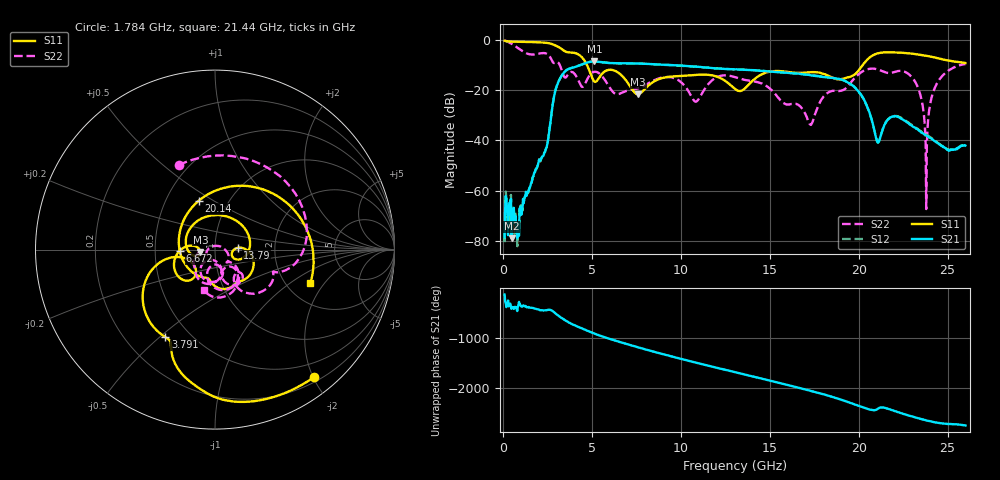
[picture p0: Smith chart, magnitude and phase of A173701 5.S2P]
!  2-Port S-parameters saved by WinCal
! VAR MeasName=S-Parameters (CALIBRATED_DATA) read from VNA (N5245A)
! VAR MeasDate=2017-6-7 10:28:45
! VAR NAME=A173701 5
! VAR FILENAME=A173701 5.S2P
! VAR DATE=2017-6-7 10:28:45
! VAR PHYS_PORTS=1,2
# Hz S DB R 50
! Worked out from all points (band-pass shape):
!   801 points, 100 MHz to 26 GHz, reference 50 ohm
!   highest |S21| = -8.61 dB at 5.151 GHz (marker M1); lowest = -79.0 dB at 488.5 MHz (marker M2)
!   |S21| within 3 dB of the highest: 3.696 GHz to 12.6 GHz (8.906 GHz wide, 109 % of centre)
!   lowest |S11| = -21.6 dB at 7.611 GHz (marker M3), VSWR 1.18, Z = 42.4 - j1.08 ohm
!   |S11| at or under -10 dB: 4.729 GHz to 20.23 GHz (15.5 GHz wide, 124 % of centre)
!   |S22| runs from -67.3 to -0.2 dB; largest |S21 - S12| = 0.0043
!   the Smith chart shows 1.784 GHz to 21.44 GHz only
!   S11 on the Smith chart (normalised r, x): 1.784 GHz: 0.27, -2.01; 3.791 GHz: 0.37, -0.52; 6.672 GHz: 0.67, -0.01; 13.79 GHz: 1.29, +0.03; 20.14 GHz: 0.73, +0.43; 21.44 GHz: 2.69, -1.47
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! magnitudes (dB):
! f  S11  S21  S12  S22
! 100 MHz  -0.3  -78.6  -80.4  -0.2
! 488.5 MHz  -0.7  -79.0  -72.6  -1.5
! 779.9 MHz  -0.8  -75.8  -73.8  -2.9
! 1.784 GHz  -0.9  -52.6  -53.1  -5.8
! 3.791 GHz  -5.0  -11.4  -11.3  -12.9
! 4.438 GHz  -6.9  -9.8  -9.8  -18.6
! 5.151 GHz  -16.6  -8.6  -8.6  -12.7
! 6.672 GHz  -14.1  -9.3  -9.3  -21.1
! 7.611 GHz  -21.6  -9.4  -9.4  -19.3
! 8.744 GHz  -15.7  -9.8  -9.8  -15.4
! 10.85 GHz  -13.9  -10.7  -10.7  -24.6
! 13.05 GHz  -19.5  -11.7  -11.7  -14.8
! 13.79 GHz  -18.0  -12.0  -11.9  -16.2
! 17.39 GHz  -12.8  -14.2  -14.1  -33.0
! 20.14 GHz  -10.8  -21.9  -22.0  -12.9
! 21.05 GHz  -5.4  -40.5  -40.6  -11.7
! 21.44 GHz  -5.0  -34.1  -34.1  -12.7
! 21.69 GHz  -4.9  -31.4  -31.3  -13.2
! 23.18 GHz  -5.7  -35.0  -34.8  -16.8
! 23.8 GHz  -6.3  -38.0  -37.8  -67.3
! 24.41 GHz  -7.2  -41.0  -40.8  -17.2
! 26 GHz  -9.2  -42.0  -41.8  -9.7
